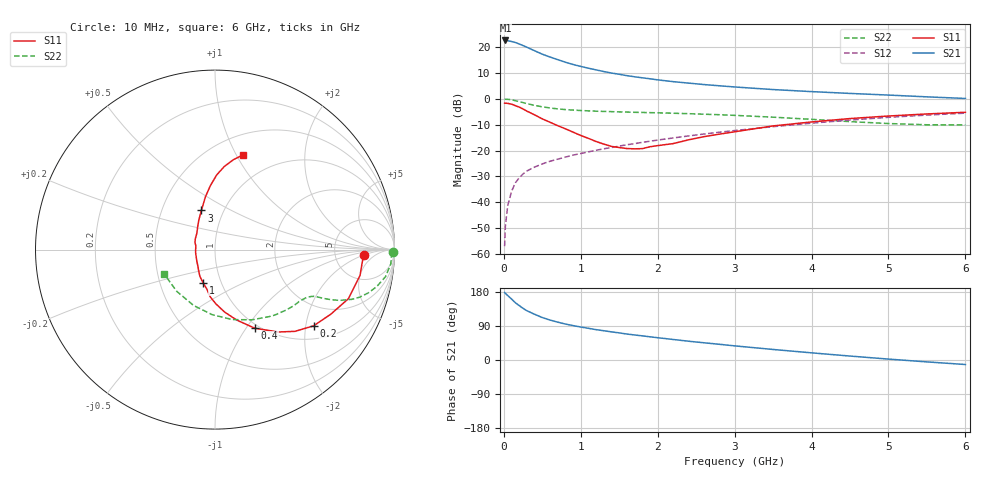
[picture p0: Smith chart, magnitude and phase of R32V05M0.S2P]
! SIEMENS Small Signal Semiconductors
! BFR181
! Si NPN RF Bipolar Junction Transistor in SOT23
! VCE = 2 V  IC = 5 mA
! Common Emitter S-Parameters:  May  1996
# GHz  S  MA  R  50
!  f  S11  S21  S12  S22
! GHz  MAG  ANG  MAG  ANG  MAG  ANG  MAG  ANG
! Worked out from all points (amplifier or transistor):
!   36 points, 10 MHz to 6 GHz, reference 50 ohm
!   highest |S21| = 22.7 dB at 20 MHz (marker M1)
!   |S21| within 3 dB of that: start of sweep to 326.8 MHz
!   unconditionally stable (mu >= 1): 1.076 GHz to 2.945 GHz
!   at 250 MHz: K = 0.42, MSG = 24.9 dB, |S12| = -29.1 dB
!   at 1.4 GHz: K = 1.06, MAG = 13.0 dB, |S12| = -18.8 dB
!   at 6 GHz: K = 0.86, MSG = 2.8 dB, |S12| = -5.5 dB
!   lowest NFmin = 1.55 dB at 450 MHz
!   S11 on the Smith chart (normalised r, x): 10 MHz: 10, -2; 200 MHz: 1.35, -2.22; 400 MHz: 0.95, -1.10; 1 GHz: 0.82, -0.31; 3 GHz: 0.79, +0.36; 6 GHz: 0.70, +1.07
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0.01  0.829 -2.1  13.5 178.0  0.0014 91.3  0.9917 -0.9
0.02  0.8246 -4.0  13.58 175.8  0.0034 87.3  0.984 -1.9
0.05  0.8207 -10.1  13.4 170.2  0.0085 85.3  0.9825 -4.7
0.1  0.7921 -20.2  12.96 160.9  0.0161 81.2  0.9622 -9.0
0.15  0.7385 -29.2  12.39 151.1  0.0237 73.7  0.9244 -12.9
0.2  0.6945 -37.7  11.6 143.6  0.0296 71.8  0.8869 -15.8
0.25  0.6374 -45.6  10.8 136.3  0.0352 68.4  0.8487 -18.2
0.3  0.5795 -52.4  10.02 130.0  0.0402 66.9  0.8106 -20.0
0.4  0.4907 -63.2  8.575 120.6  0.0478 63.8  0.7491 -22.2
0.5  0.4105 -72.9  7.356 112.0  0.055 62.5  0.7022 -23.4
0.6  0.3531 -81.1  6.487 105.4  0.0619 62.2  0.6677 -24.1
0.8  0.2637 -95.9  5.143 94.9  0.0745 62.5  0.6216 -24.9
1  0.1955 -110.0  4.262 87.0  0.0874 63.4  0.596 -26.0
1.1  0.1718 -119.3  3.935 83.6  0.0942 63.5  0.5865 -26.7
1.3  0.133 -135.8  3.387 77.2  0.108 63.9  0.5719 -28.1
1.6  0.1091 -171.6  2.825 68.5  0.1293 64.1  0.5556 -30.8
2.2  0.136 138.1  2.162 54.2  0.175 62.6  0.5278 -38.2
3  0.2307 109.2  1.704 37.3  0.2439 57.9  0.4798 -51.1
3.5  0.2996 100.2  1.518 27.8  0.29 53.8  0.4426 -62.1
4.5  0.4162 88.7  1.277 10.4  0.3894 43.4  0.3628 -92.5
5.5  0.511 78.5  1.096 -5.0  0.4863 30.5  0.3154 -132.5
6  0.5506 73.4  1.02 -11.9  0.53 23.4  0.3138 -154.2
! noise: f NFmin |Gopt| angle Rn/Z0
0.45  1.55  0.48  17  0.36
0.9  1.65  0.4  35  0.34
1.8  2  0.18  88  0.34
